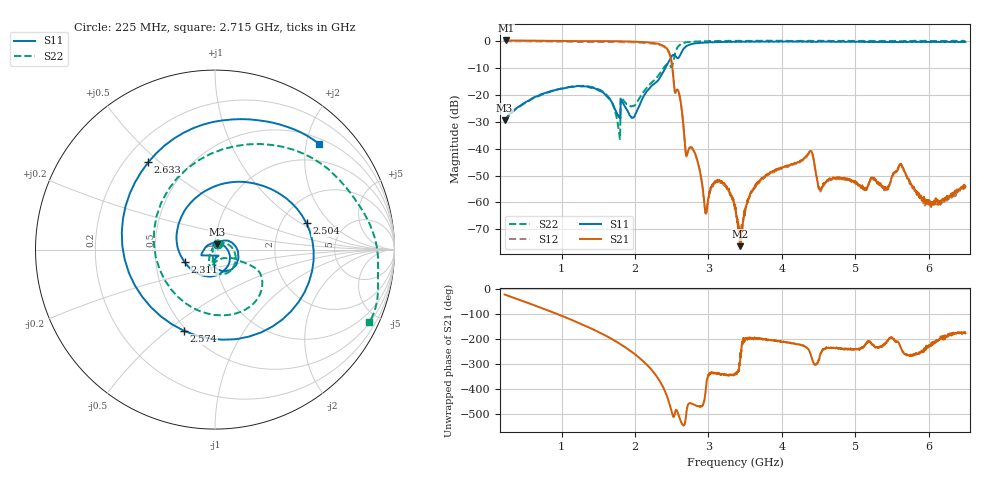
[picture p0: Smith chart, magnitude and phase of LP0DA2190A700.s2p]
!Agilent Technologies,E8358A,US41080443,A.07.50.56
!Agilent E8358A: A.07.50.56
!Date: Wednesday, July 06, 2016 14:47:11
!Correction: S11(Full 2 Port(1,2))
!S21(Full 2 Port(1,2))
!S12(Full 2 Port(1,2))
!S22(Full 2 Port(1,2))
!S2P File: Measurements: S11, S21, S12, S22:
# Hz S  dB  R 50
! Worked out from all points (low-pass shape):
!   1601 points, 225 MHz to 6.5 GHz, reference 50 ohm
!   highest |S21| = 0.23 dB at 240.7 MHz (marker M1); lowest = -76.3 dB at 3.433 GHz (marker M2)
!   |S21| within 3 dB of the highest: start of sweep to 2.433 GHz
!   lowest |S11| = -29.5 dB at 225 MHz (marker M3), VSWR 1.07, Z = 51 + j3.23 ohm
!   |S11| at or under -10 dB: start of sweep to 2.414 GHz
!   |S22| runs from -36.4 to 0.2 dB; largest |S21 - S12| = 0.039
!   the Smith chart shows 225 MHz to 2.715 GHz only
!   S11 on the Smith chart (normalised r, x): 225 MHz: 1.02, +0.06; 2.311 GHz: 0.70, -0.10; 2.504 GHz: 2.75, +1.12; 2.574 GHz: 0.48, -0.57; 2.633 GHz: 0.30, +0.46; 2.715 GHz: 0.61, +2.26
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2.25e8  -29.49 70.8  0.22 -23.9  -0.11 -23.8  -29.75 62.5
2.406875e8  -29.03 69.9  0.23 -25.5  -0.10 -25.4  -29.12 60.6
7.8975e8  -19.18 14.7  0.10 -84.5  -0.23 -84.3  -19.38 -4.7
1.272141e9  -16.90 -42.6  -0.01 -141.8  -0.34 -141.7  -16.63 -61.4
1.656484e9  -21.66 -91.6  -0.05 163.4  -0.38 163.5  -21.40 -113.1
1.985922e9  -28.35 73.5  -0.20 101.1  -0.53 101.2  -24.03 -52.8
2.311438e9  -14.75 -157.5  -0.99 2.9  -1.31 3.0  -13.08 -24.1
2.319281e9  -14.51 -164.3  -1.04 -0.6  -1.36 -0.6  -12.80 -24.2
2.429094e9  -9.22 93.1  -2.66 -63.9  -2.96 -63.9  -8.74 -51.8
2.503609e9  -5.51 16.0  -8.59 -136.7  -8.95 -136.6  -9.56 -172.7
2.574203e9  -6.30 -110.9  -18.02 -128.7  -18.30 -128.6  -2.56 43.1
2.633031e9  -4.26 127.3  -24.58 -175.2  -24.85 -175.4  -0.96 3.3
2.715391e9  -1.65 45.3  -41.61 -109.8  -42.01 -109.5  -0.43 -25.2
2.962469e9  -0.52 -36.7  -64.13 -49.3  -63.76 -46.3  -0.04 -62.0
3.138953e9  -0.32 -63.6  -51.99 21.6  -52.47 21.6  0.07 -75.3
3.3625e9  -0.32 -87.9  -61.74 20.0  -62.13 22.8  0.03 -88.0
3.433094e9  -0.32 -93.9  -76.28 71.4  -72.14 108.6  0.04 -91.1
3.668406e9  -0.16 -111.4  -52.59 162.4  -53.10 160.4  0.12 -99.8
4.409641e9  -0.34 -155.6  -41.36 82.2  -41.60 82.3  0.02 -120.0
4.523375e9  -0.22 -162.4  -55.24 96.3  -55.80 89.6  0.09 -122.5
5.456781e9  -0.38 136.7  -54.15 160.6  -54.05 158.0  0.01 -146.2
6.5e9  -0.32 70.6  -54.07 -178.8  -54.86 -176.4  0.02 -178.1
